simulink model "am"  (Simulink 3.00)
settings: Solver=ode45  StartTime=0.0  StopTime=10.0  RelTol=1e-3
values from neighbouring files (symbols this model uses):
  J = 0.0017    [Data.m]
  kr = Lm/Lr    (= 0.963591022444)    [Data.m]
  Lm = .5796    (= 0.5796)    [Data.m]
  Ls1 = Ls-Lm^2/Lr    (= 0.0430026433915)    [Data.m]
  p = 1    [Data.m]
  R1 = Rs+kr^2*Rr    (= 11.0434783366)    [Data.m]
  T1 = Ls1/R1    (= 0.00389394012293)    [Data.m]
  Tr = Lr/Rr    (= 0.162567567568)    [Data.m]
undefined symbols (not defined in the file or in its folder): km
libraries: simulink_extras x1

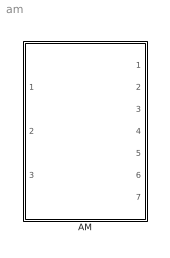
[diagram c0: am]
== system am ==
  AM : Subsystem

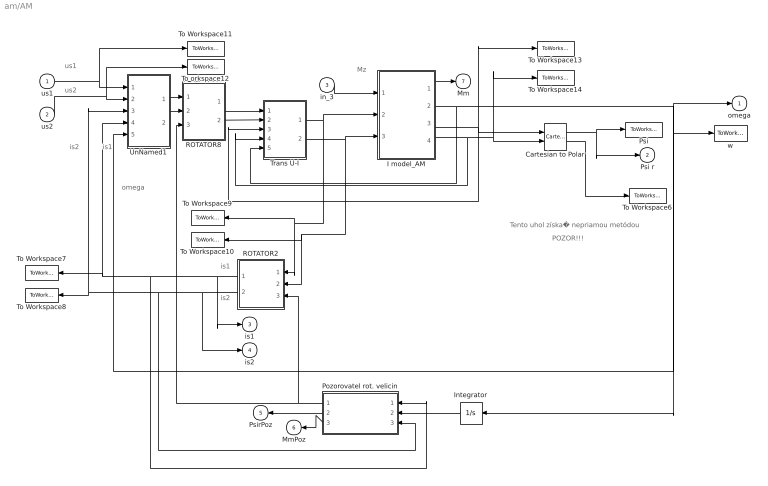
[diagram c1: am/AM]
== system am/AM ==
  note: is2
  note: is1
  note: omega
  note: us2
  note: us1
  note: Mz
  note: is1
  note: is2
  note: POZOR!!!
  note: Tento uhol získa� nepriamou metódou
  us1 : Inport  Port=1  PortWidth=-1  SampleTime=-1  DataType=auto
  us2 : Inport  Port=2  PortWidth=-1  SampleTime=-1  DataType=auto
  in_3 : Inport  Port=3  PortWidth=-1  SampleTime=-1  DataType=auto
  Cartesian to Polar : simulink_extras/Transformations/Cartesian to Polar
  I model_AM : Subsystem
  Integrator : Integrator  Orientation=left  ExternalReset=none  InitialConditionSource=internal  InitialCondition=0  LimitOutput=off  UpperSaturationLimit=inf  LowerSaturationLimit=-inf  ShowSaturationPort=off  ShowStatePort=off  AbsoluteTolerance=auto
  Pozorovatel rot. velicin : Subsystem  Orientation=left
  Psi : ToWorkspace  VariableName=Psi  SampleTime=0  SaveFormat=Matrix
  ROTATOR2 : Subsystem  Orientation=left
  ROTATOR8 : Subsystem
  To Workspace10 : ToWorkspace  VariableName=isb  SampleTime=0  SaveFormat=Matrix
  To Workspace11 : ToWorkspace  VariableName=us1  SampleTime=0  SaveFormat=Matrix
  To Workspace13 : ToWorkspace  VariableName=psiral  SampleTime=0  SaveFormat=Matrix
  To Workspace14 : ToWorkspace  VariableName=psirbe  SampleTime=0  SaveFormat=Matrix
  To Workspace6 : ToWorkspace  VariableName=theta  SampleTime=0  SaveFormat=Matrix
  To Workspace7 : ToWorkspace  VariableName=is1  SampleTime=0  SaveFormat=Matrix
  To Workspace8 : ToWorkspace  VariableName=is2  SampleTime=0  SaveFormat=Matrix
  To Workspace9 : ToWorkspace  VariableName=isal  SampleTime=0  SaveFormat=Matrix
  To orkspace12 : ToWorkspace  VariableName=us2  SampleTime=0  SaveFormat=Matrix
  Trans U-I : Subsystem
  UnNamed1 : Subsystem
  w : ToWorkspace  VariableName=omega  SampleTime=0  SaveFormat=Matrix
  omega : Outport  Port=1  InitialOutput=0
  Psi r : Outport  Port=2  InitialOutput=0
  is1 : Outport  Port=3  InitialOutput=0
  is2 : Outport  Port=4  InitialOutput=0
  PsirPoz : Outport  Orientation=left  Port=5  InitialOutput=0
  MmPoz : Outport  Orientation=left  Port=6  InitialOutput=0
  Mm : Outport  Port=7  InitialOutput=0
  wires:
  UnNamed1/2(Outport2) -> ROTATOR8/2(in_2)
  UnNamed1/1(Outport1) -> ROTATOR8/1(in_1)
  Trans U-I/2(out_2) -> I model_AM/3(isbe), To Workspace10/1, ROTATOR2/2(in_2)
  ROTATOR8/2(out_2) -> Trans U-I/2(in_2)
  ROTATOR8/1(out_1) -> Trans U-I/1(in_1)
  in_3/1 -> I model_AM/1(Mz)
  Trans U-I/1(out_1) -> I model_AM/2(isal), To Workspace9/1, ROTATOR2/1(in_1)
  ROTATOR2/1(out_1) -> is1/1, UnNamed1/4(in_6), To Workspace7/1, Pozorovatel rot. velicin/1(Is1)
  ROTATOR2/2(out_2) -> is2/1, UnNamed1/3(in_3), To Workspace8/1, Pozorovatel rot. velicin/3(Is2)
  us1/1 -> UnNamed1/1(in_1), To Workspace11/1
  us2/1 -> UnNamed1/2(in_2), To orkspace12/1
  Pozorovatel rot. velicin/1(ThetaPoz) -> ROTATOR8/3(in_3), ROTATOR2/3(in_3)
  Pozorovatel rot. velicin/2(PsirPoz) -> PsirPoz/1
  Pozorovatel rot. velicin/3(MmPoz) -> MmPoz/1
  Integrator/1 -> Pozorovatel rot. velicin/2(theta)
  Cartesian to Polar/1 -> Psi/1, Psi r/1
  Cartesian to Polar/2 -> To Workspace6/1
  I model_AM/1(Mm) -> Mm/1
  I model_AM/3(Psir_al) -> Cartesian to Polar/1, To Workspace13/1, Trans U-I/3(in_6)
  I model_AM/4(Psir_be) -> Cartesian to Polar/2, To Workspace14/1, Trans U-I/4(in_4)
  I model_AM/2(omega) -> UnNamed1/5(in_5), omega/1, w/1, Integrator/1, Trans U-I/5(in_8)

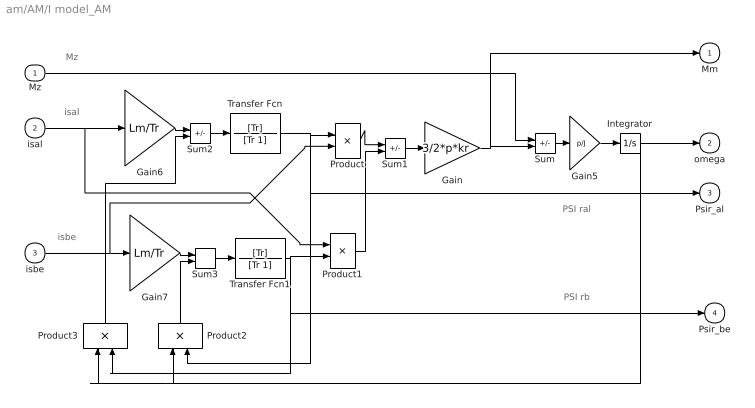
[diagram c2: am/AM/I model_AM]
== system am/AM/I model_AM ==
  note: isal
  note: PSI ral
  note: isbe
  note: PSI rb
  note: Mz
  Mz : Inport  Port=1  PortWidth=-1  SampleTime=-1  DataType=auto
  isal : Inport  Port=2  PortWidth=-1  SampleTime=-1  DataType=auto
  isbe : Inport  Port=3  PortWidth=-1  SampleTime=-1  DataType=auto
  Gain : Gain  Gain=3/2*p*kr  SaturateOnIntegerOverflow=on
  Gain5 : Gain  Gain=p/J  SaturateOnIntegerOverflow=on
  Gain6 : Gain  Gain=Lm/Tr  SaturateOnIntegerOverflow=on
  Gain7 : Gain  Gain=Lm/Tr  SaturateOnIntegerOverflow=on
  Integrator : Integrator  ExternalReset=none  InitialConditionSource=internal  InitialCondition=0  LimitOutput=off  UpperSaturationLimit=inf  LowerSaturationLimit=-inf  ShowSaturationPort=off  ShowStatePort=off  AbsoluteTolerance=auto
  Product : Product  Inputs=2  SaturateOnIntegerOverflow=on
  Product1 : Product  Inputs=2  SaturateOnIntegerOverflow=on
  Product2 : Product  Orientation=up  Inputs=2  SaturateOnIntegerOverflow=on
  Product3 : Product  Orientation=up  Inputs=2  SaturateOnIntegerOverflow=on
  Sum : Sum  Inputs=-+  SaturateOnIntegerOverflow=on
  Sum1 : Sum  Inputs=+-  SaturateOnIntegerOverflow=on
  Sum2 : Sum  Inputs=+-  SaturateOnIntegerOverflow=on
  Sum3 : Sum  Inputs=++  SaturateOnIntegerOverflow=on
  Transfer Fcn : TransferFcn  Numerator=[Tr]  Denominator=[Tr 1]
  Transfer Fcn1 : TransferFcn  Numerator=[Tr]  Denominator=[Tr 1]
  Mm : Outport  Port=1  InitialOutput=0
  omega : Outport  Port=2  InitialOutput=0
  Psir_al : Outport  Port=3  InitialOutput=0
  Psir_be : Outport  Port=4  InitialOutput=0
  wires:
  Gain/1 -> Mm/1, Sum/2
  Product1/1 -> Sum1/2
  Mz/1 -> Sum/1
  isbe/1 -> Gain7/1, Product/2
  Product2/1 -> Sum3/2
  Sum3/1 -> Transfer Fcn1/1
  Sum2/1 -> Transfer Fcn/1
  Product/1 -> Sum1/1
  Sum1/1 -> Gain/1
  Sum/1 -> Gain5/1
  Integrator/1 -> omega/1, Product3/1, Product2/1
  Transfer Fcn/1 -> Product/1, Product2/2, Psir_al/1
  Gain7/1 -> Sum3/1
  Gain6/1 -> Sum2/1
  Transfer Fcn1/1 -> Product1/2, Product3/2, Psir_be/1
  Product3/1 -> Sum2/2
  isal/1 -> Gain6/1, Product1/1
  Gain5/1 -> Integrator/1

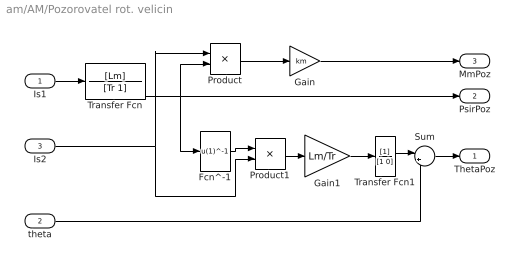
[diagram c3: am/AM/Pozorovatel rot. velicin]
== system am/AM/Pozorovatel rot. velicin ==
  Is1 : Inport  Port=1  PortWidth=-1  SampleTime=-1  DataType=auto
  theta : Inport  Port=2  PortWidth=-1  SampleTime=-1  DataType=auto
  Is2 : Inport  Port=3  PortWidth=-1  SampleTime=-1  DataType=auto
  Fcn^-1 : Fcn  Expr=u(1)^-1
  Gain : Gain  Gain=km  SaturateOnIntegerOverflow=on
  Gain1 : Gain  Gain=Lm/Tr  SaturateOnIntegerOverflow=on
  Product : Product  Inputs=2  SaturateOnIntegerOverflow=on
  Product1 : Product  Inputs=2  SaturateOnIntegerOverflow=on
  Sum : Sum  Inputs=|++  SaturateOnIntegerOverflow=on
  Transfer Fcn : TransferFcn  Numerator=[Lm]  Denominator=[Tr 1]
  Transfer Fcn1 : TransferFcn  Numerator=[1]  Denominator=[1 0]
  ThetaPoz : Outport  Port=1
  PsirPoz : Outport  Port=2
  MmPoz : Outport  Port=3
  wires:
  Is1/1 -> Transfer Fcn/1
  Transfer Fcn1/1 -> Sum/1
  theta/1 -> Sum/2
  Sum/1 -> ThetaPoz/1
  Transfer Fcn/1 -> PsirPoz/1, Product/2, Fcn^-1/1
  Gain/1 -> MmPoz/1
  Product/1 -> Gain/1
  Gain1/1 -> Transfer Fcn1/1
  Is2/1 -> Product/1, Product1/2
  Fcn^-1/1 -> Product1/1
  Product1/1 -> Gain1/1

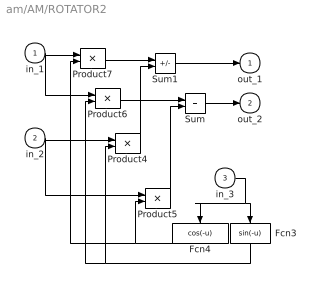
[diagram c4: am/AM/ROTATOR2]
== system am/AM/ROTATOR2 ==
  in_1 : Inport  Port=1  PortWidth=-1  SampleTime=-1  DataType=auto
  in_2 : Inport  Port=2  PortWidth=-1  SampleTime=-1  DataType=auto
  in_3 : Inport  Port=3  PortWidth=-1  SampleTime=-1  DataType=auto
  Fcn3 : Fcn  Orientation=down  Expr=sin(-u)
  Fcn4 : Fcn  Orientation=down  Expr=cos(-u)
  Product{4..7} (4 alike) : Product  Inputs=2  SaturateOnIntegerOverflow=on
  Sum : Sum  Inputs=++  SaturateOnIntegerOverflow=on
  Sum1 : Sum  Inputs=+-  SaturateOnIntegerOverflow=on
  out_1 : Outport  Port=1  InitialOutput=0
  out_2 : Outport  Port=2  InitialOutput=0
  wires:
  in_3/1 -> Fcn3/1, Fcn4/1
  in_2/1 -> Product5/1, Product4/1
  Sum/1 -> out_2/1
  Sum1/1 -> out_1/1
  in_1/1 -> Product6/1, Product7/1
  Product4/1 -> Sum1/2
  Product7/1 -> Sum1/1
  Fcn3/1 -> Product4/2, Product6/2
  Product6/1 -> Sum/1
  Product5/1 -> Sum/2
  Fcn4/1 -> Product7/2, Product5/2

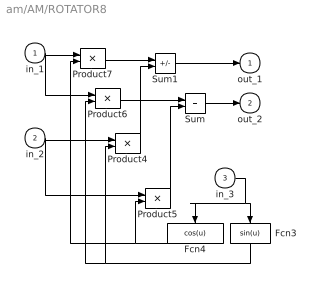
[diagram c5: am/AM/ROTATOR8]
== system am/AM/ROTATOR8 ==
  in_1 : Inport  Port=1  PortWidth=-1  SampleTime=-1  DataType=auto
  in_2 : Inport  Port=2  PortWidth=-1  SampleTime=-1  DataType=auto
  in_3 : Inport  Port=3  PortWidth=-1  SampleTime=-1  DataType=auto
  Fcn3 : Fcn  Orientation=down  Expr=sin(u)
  Fcn4 : Fcn  Orientation=down  Expr=cos(u)
  Product{4..7} (4 alike) : Product  Inputs=2  SaturateOnIntegerOverflow=on
  Sum : Sum  Inputs=++  SaturateOnIntegerOverflow=on
  Sum1 : Sum  Inputs=+-  SaturateOnIntegerOverflow=on
  out_1 : Outport  Port=1  InitialOutput=0
  out_2 : Outport  Port=2  InitialOutput=0
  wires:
  Fcn4/1 -> Product7/2, Product5/2
  Product5/1 -> Sum/2
  Product6/1 -> Sum/1
  Fcn3/1 -> Product4/2, Product6/2
  Product7/1 -> Sum1/1
  Product4/1 -> Sum1/2
  in_1/1 -> Product7/1, Product6/1
  Sum1/1 -> out_1/1
  Sum/1 -> out_2/1
  in_2/1 -> Product4/1, Product5/1
  in_3/1 -> Fcn3/1, Fcn4/1

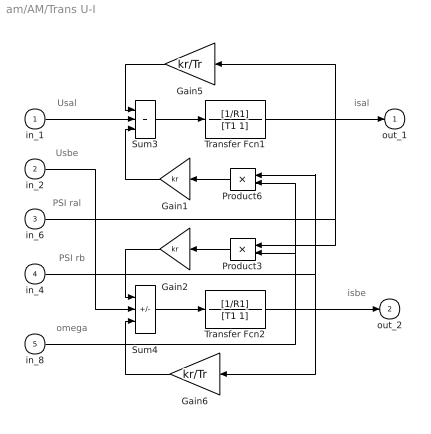
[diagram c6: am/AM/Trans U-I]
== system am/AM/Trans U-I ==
  note: PSI rb
  note: PSI ral
  note: omega
  note: Usal
  note: Usbe
  note: isal
  note: isbe
  in_1 : Inport  Port=1  PortWidth=-1  SampleTime=-1  DataType=auto
  in_2 : Inport  Port=2  PortWidth=-1  SampleTime=-1  DataType=auto
  in_6 : Inport  Port=3  PortWidth=-1  SampleTime=-1  DataType=auto
  in_4 : Inport  Port=4  PortWidth=-1  SampleTime=-1  DataType=auto
  in_8 : Inport  Port=5  PortWidth=-1  SampleTime=-1  DataType=auto
  Gain1 : Gain  Orientation=left  Gain=kr  SaturateOnIntegerOverflow=on
  Gain2 : Gain  Orientation=left  Gain=kr  SaturateOnIntegerOverflow=on
  Gain5 : Gain  Orientation=left  Gain=kr/Tr  SaturateOnIntegerOverflow=on
  Gain6 : Gain  Orientation=left  Gain=kr/Tr  SaturateOnIntegerOverflow=on
  Product3 : Product  Orientation=left  Inputs=2  SaturateOnIntegerOverflow=on
  Product6 : Product  Orientation=left  Inputs=2  SaturateOnIntegerOverflow=on
  Sum3 : Sum  Inputs=+++  SaturateOnIntegerOverflow=on
  Sum4 : Sum  Inputs=-++  SaturateOnIntegerOverflow=on
  Transfer Fcn1 : TransferFcn  Numerator=[1/R1]  Denominator=[T1 1]
  Transfer Fcn2 : TransferFcn  Numerator=[1/R1]  Denominator=[T1 1]
  out_1 : Outport  Port=1  InitialOutput=0
  out_2 : Outport  Port=2  InitialOutput=0
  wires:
  in_2/1 -> Sum4/2
  Gain1/1 -> Sum3/3
  Gain2/1 -> Sum4/1
  Transfer Fcn2/1 -> out_2/1
  Transfer Fcn1/1 -> out_1/1
  Sum3/1 -> Transfer Fcn1/1
  Sum4/1 -> Transfer Fcn2/1
  Gain6/1 -> Sum4/3
  Gain5/1 -> Sum3/1
  in_1/1 -> Sum3/2
  Product6/1 -> Gain1/1
  Product3/1 -> Gain2/1
  in_8/1 -> Product6/2, Product3/2
  in_6/1 -> Product3/1, Gain5/1
  in_4/1 -> Gain6/1, Product6/1

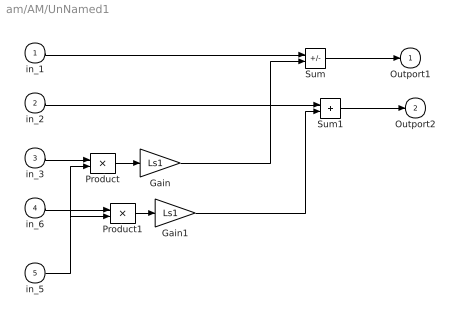
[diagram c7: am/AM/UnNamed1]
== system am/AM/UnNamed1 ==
  in_1 : Inport  Port=1  PortWidth=-1  SampleTime=-1  DataType=auto
  in_2 : Inport  Port=2  PortWidth=-1  SampleTime=-1  DataType=auto
  in_3 : Inport  Port=3  PortWidth=-1  SampleTime=-1  DataType=auto
  in_6 : Inport  Port=4  PortWidth=-1  SampleTime=-1  DataType=auto
  in_5 : Inport  Port=5  PortWidth=-1  SampleTime=-1  DataType=auto
  Gain : Gain  Gain=Ls1  SaturateOnIntegerOverflow=on
  Gain1 : Gain  Gain=Ls1  SaturateOnIntegerOverflow=on
  Product : Product  Inputs=2  SaturateOnIntegerOverflow=on
  Product1 : Product  Inputs=2  SaturateOnIntegerOverflow=on
  Sum : Sum  Inputs=+-  SaturateOnIntegerOverflow=on
  Sum1 : Sum  Inputs=++  SaturateOnIntegerOverflow=on
  Outport1 : Outport  Port=1  InitialOutput=0
  Outport2 : Outport  Port=2  InitialOutput=0
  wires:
  Sum1/1 -> Outport2/1
  in_2/1 -> Sum1/1
  Gain1/1 -> Sum1/2
  Product1/1 -> Gain1/1
  in_5/1 -> Product/2, Product1/2
  in_6/1 -> Product1/1
  Sum/1 -> Outport1/1
  Gain/1 -> Sum/2
  in_1/1 -> Sum/1
  Product/1 -> Gain/1
  in_3/1 -> Product/1
